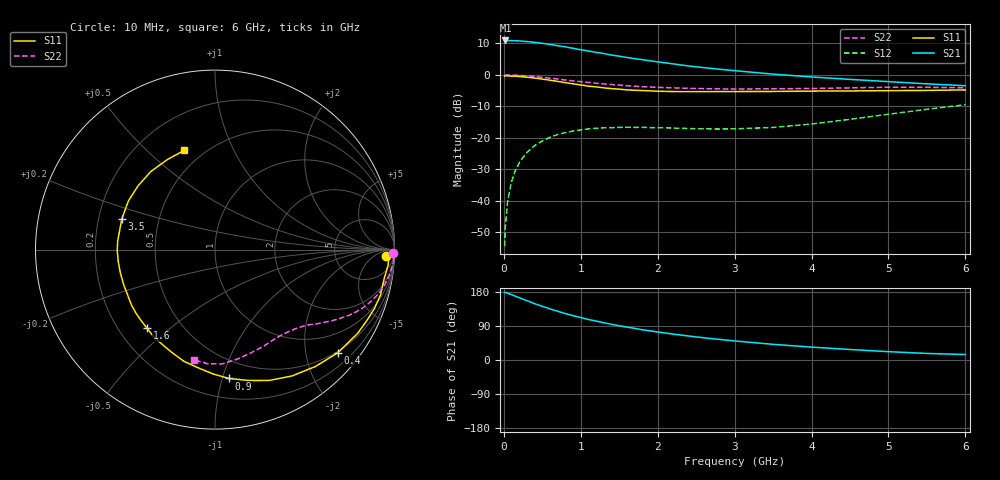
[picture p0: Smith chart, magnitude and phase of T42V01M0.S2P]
! Infineon Technologies  Discrete & RF Semiconductors
! BFR182T
! Si NPN RF Bipolar Junction Transistor in SC75
! VCE = 2 V  IC = 1 mA
! Common Emitter S-Parameters:  October  1999
# GHz  S  MA  R  50
!  f  S11  S21  S12  S22
! GHz  MAG  ANG  MAG  ANG  MAG  ANG  MAG  ANG
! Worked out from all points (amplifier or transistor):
!   36 points, 10 MHz to 6 GHz, reference 50 ohm
!   highest |S21| = 11.0 dB at 20 MHz (marker M1)
!   |S21| within 3 dB of that: start of sweep to 1.01 GHz
!   unconditionally stable (mu >= 1): 2.364 GHz to 4.599 GHz
!   at 250 MHz: K = 0.09, MSG = 18.4 dB, |S12| = -26.2 dB
!   at 1.4 GHz: K = 0.59, MSG = 11.5 dB, |S12| = -16.8 dB
!   at 6 GHz: K = 0.85, MSG = 3.0 dB, |S12| = -9.5 dB
!   S11 on the Smith chart (normalised r, x): 10 MHz: 26, -20; 400 MHz: 0.47, -2.67; 900 MHz: 0.35, -1.05; 1.6 GHz: 0.32, -0.42; 3.5 GHz: 0.30, +0.15; 6 GHz: 0.40, +0.66
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0.01  0.9526 -2.1  3.492 178.7  0.0019 87.0  0.9915 -1.2
0.02  0.9745 -0.8  3.533 178.8  0.0039 88.3  0.9904 -0.7
0.05  0.9678 -5.3  3.522 176.1  0.01 89.1  0.9969 -2.0
0.1  0.9563 -9.9  3.502 172.5  0.0203 84.5  0.9961 -4.1
0.15  0.9561 -15.4  3.496 168.4  0.0302 80.5  0.9887 -6.0
0.25  0.9336 -25.1  3.433 160.5  0.0491 75.4  0.9749 -9.9
0.4  0.8933 -40.1  3.298 148.7  0.0752 66.7  0.9421 -15.3
0.5  0.8587 -49.3  3.184 141.8  0.0893 61.7  0.9162 -18.3
0.6  0.8247 -58.6  3.055 134.8  0.1022 57.1  0.8877 -21.3
0.8  0.7537 -75.4  2.794 122.6  0.121 48.7  0.8315 -26.1
0.9  0.7225 -83.7  2.651 117.0  0.1286 45.4  0.8044 -28.1
1.1  0.6642 -98.5  2.405 106.9  0.1389 39.7  0.7589 -31.6
1.3  0.6232 -112.2  2.189 98.3  0.1445 35.5  0.7189 -34.6
1.4  0.6057 -118.5  2.07 94.2  0.1453 33.5  0.704 -36.0
1.6  0.579 -130.7  1.894 86.6  0.1471 31.0  0.674 -38.3
1.8  0.5645 -141.6  1.75 79.8  0.147 29.5  0.6511 -40.9
2.2  0.5449 -158.9  1.5 68.3  0.1433 29.1  0.6241 -45.6
2.8  0.5446 -179.3  1.234 54.4  0.1383 33.7  0.6008 -53.9
3.5  0.5466 161.9  1.03 41.3  0.1464 44.8  0.6025 -63.5
4.5  0.5567 140.3  0.85 27.7  0.1969 57.3  0.623 -78.6
5.5  0.5675 117.9  0.722 17.3  0.2851 59.0  0.637 -93.8
6  0.5789 107.3  0.674 14.5  0.3365 56.3  0.6257 -101.0
